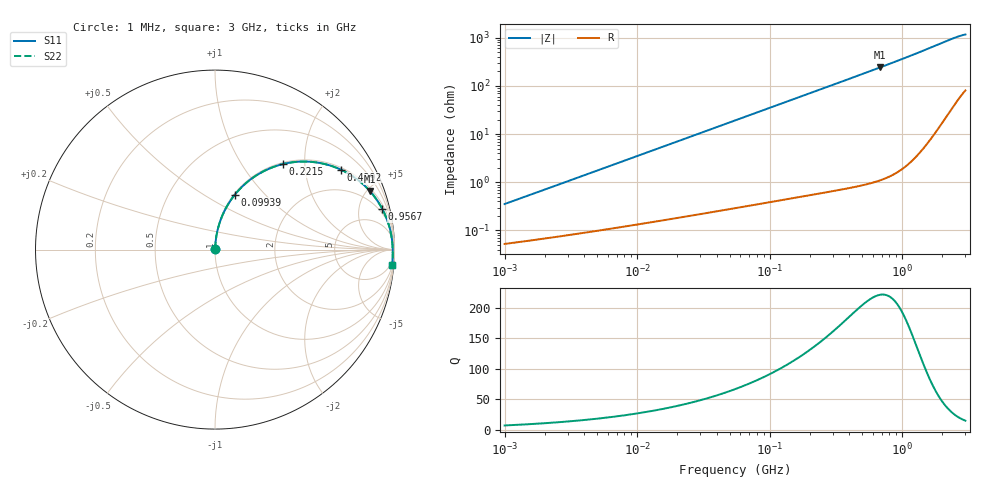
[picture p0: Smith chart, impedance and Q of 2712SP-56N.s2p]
# MHz  S  MA  R  50
!Freq  MagS11  AngS11  MagS21  AngS21  MagS12  AngS12  MagS22  AngS22
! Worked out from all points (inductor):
!   801 points, 1 MHz to 3 GHz, reference 50 ohm
!   read as one part in series: L = 55.8 nH near 1.041 MHz
!   highest Q = 221 at 680.5 MHz (marker M1), where L = 56.7 nH
!   S11 on the Smith chart (normalised r, x): 1 MHz: 1.00, +0.01; 99.39 MHz: 1.01, +0.69; 221.5 MHz: 1.03, +1.56; 429.2 MHz: 1.08, +3.10; 956.7 MHz: 1.42, +8.06; 3 GHz: 2, -22
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1  0.003519 81.2  0.9995 -0.2  0.9995 -0.2  0.003519 81.2
3.829105  0.01335 85.4  0.999 -0.8  0.999 -0.8  0.01335 85.4
14.51587  0.05042 85.3  0.9972 -2.9  0.9972 -2.9  0.05042 85.3
29.86408  0.1032 82.8  0.9925 -6.0  0.9925 -6.0  0.1032 82.8
55.02866  0.1877 78.2  0.9794 -11.0  0.9794 -11.0  0.1877 78.2
75.82913  0.2545 74.3  0.9638 -14.9  0.9638 -14.9  0.2545 74.3
99.38614  0.326 70.1  0.9418 -19.3  0.9418 -19.3  0.326 70.1
143.9893  0.4468 62.6  0.8906 -26.9  0.8906 -26.9  0.4468 62.6
208.6098  0.5862 53.2  0.8058 -36.4  0.8058 -36.4  0.5861 53.2
221.5356  0.6093 51.5  0.7885 -38.1  0.7885 -38.1  0.6092 51.5
262.6749  0.6736 46.6  0.7347 -43.0  0.7347 -43.0  0.6735 46.6
308.3487  0.7307 41.9  0.6783 -47.7  0.6783 -47.7  0.7306 41.9
361.9643  0.7827 37.3  0.6181 -52.4  0.6181 -52.4  0.7825 37.3
429.1813  0.8308 32.4  0.5523 -57.3  0.5523 -57.3  0.8307 32.4
540.4116  0.8834 26.3  0.4646 -63.4  0.4646 -63.4  0.8832 26.3
680.4692  0.9222 20.8  0.3829 -69.0  0.3829 -69.0  0.922 20.8
790.8254  0.941 17.5  0.3343 -72.2  0.3343 -72.2  0.9408 17.5
956.6621  0.959 13.7  0.2789 -76.0  0.2789 -76.0  0.9588 13.7
1279.238  0.9768 8.6  0.2075 -81.0  0.2075 -81.0  0.9766 8.6
1762.781  0.9871 3.6  0.1461 -85.5  0.1461 -85.5  0.9869 3.6
2528.433  0.9909 -2.0  0.09761 -89.6  0.09761 -89.6  0.9908 -2.0
3000  0.9903 -5.1  0.08449 -91.1  0.08449 -91.1  0.9903 -5.1
